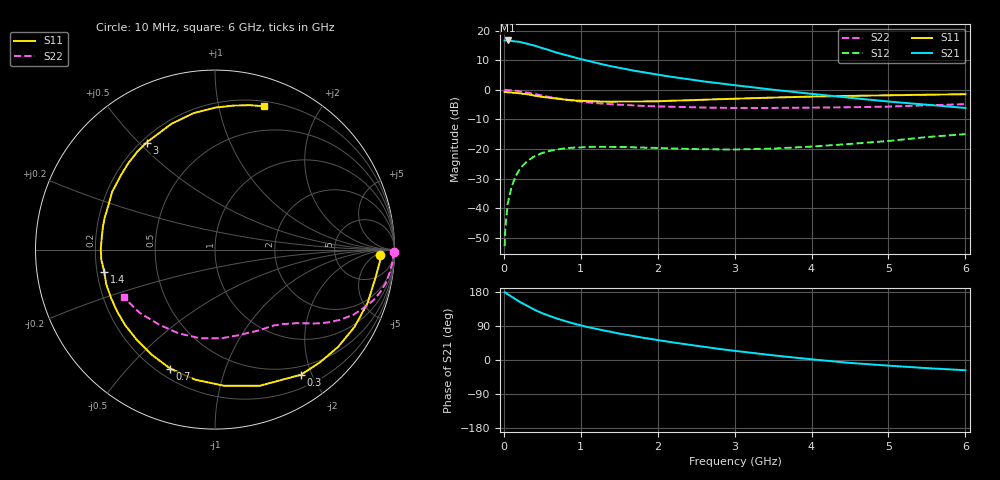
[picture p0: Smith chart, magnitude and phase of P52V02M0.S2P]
! SIEMENS Small Signal Semiconductors
! BFP183
! Si NPN RF Bipolar Junction Transistor in SOT143
! VCE = 2 V  IC = 2 mA
! Common Emitter S-Parameters:  March  1996
# GHz  S  MA  R  50
!  f  S11  S21  S12  S22
! GHz  MAG  ANG  MAG  ANG  MAG  ANG  MAG  ANG
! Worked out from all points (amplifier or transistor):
!   36 points, 10 MHz to 6 GHz, reference 50 ohm
!   highest |S21| = 16.7 dB at 50 MHz (marker M1)
!   |S21| within 3 dB of that: start of sweep to 554.7 MHz
!   unconditionally stable (mu >= 1): 2.078 GHz to 5.998 GHz
!   at 250 MHz: K = 0.12, MSG = 20.7 dB, |S12| = -25.4 dB
!   at 1.4 GHz: K = 0.68, MSG = 13.6 dB, |S12| = -19.3 dB
!   at 6 GHz: K = 1.00, MSG = 4.4 dB, |S12| = -15.0 dB
!   S11 on the Smith chart (normalised r, x): 10 MHz: 20, -8; 300 MHz: 0.38, -1.84; 700 MHz: 0.25, -0.66; 1.4 GHz: 0.23, -0.09; 3 GHz: 0.22, +0.53; 6 GHz: 0.25, +1.37
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0.01  0.9183 -1.9  6.817 179.0  0.0023 82.7  0.9991 -0.7
0.02  0.9215 -4.0  6.808 178.0  0.0048 85.3  0.9936 -1.5
0.05  0.908 -9.9  6.819 173.6  0.012 87.2  0.9922 -3.7
0.1  0.9007 -19.3  6.692 167.1  0.0229 78.1  0.9815 -7.5
0.2  0.8742 -38.3  6.477 154.3  0.0444 68.9  0.9507 -14.4
0.25  0.8582 -47.1  6.23 148.5  0.0534 64.0  0.9279 -17.6
0.3  0.8459 -55.5  6.009 143.4  0.062 59.3  0.9009 -20.3
0.4  0.7986 -71.8  5.574 132.5  0.0761 51.1  0.8528 -25.2
0.5  0.7602 -86.2  5.067 123.4  0.0861 44.0  0.7993 -29.3
0.6  0.7331 -98.7  4.638 115.8  0.0938 38.1  0.7547 -32.4
0.7  0.7082 -110.6  4.2 108.8  0.0989 33.4  0.7172 -34.9
0.8  0.6836 -121.0  3.883 102.4  0.1032 29.3  0.6854 -36.9
0.9  0.6657 -130.7  3.585 96.7  0.1058 25.9  0.6565 -38.7
1.1  0.6451 -147.8  3.079 86.4  0.1087 20.2  0.6129 -41.9
1.4  0.6292 -168.7  2.496 74.0  0.109 14.0  0.5733 -46.3
1.8  0.6371 168.5  2 59.1  0.1061 10.4  0.536 -51.9
2.2  0.6569 150.8  1.643 46.4  0.1027 8.9  0.518 -58.4
3  0.7081 122.6  1.199 24.2  0.0985 12.6  0.495 -74.4
3.5  0.7409 109.3  1.005 12.3  0.1021 16.8  0.4954 -85.7
4.5  0.7914 89.8  0.735 -7.7  0.1222 22.8  0.5089 -113.3
5.5  0.8275 76.5  0.561 -21.5  0.1598 23.0  0.5482 -140.0
6  0.8442 71.1  0.495 -27.0  0.1788 19.6  0.5737 -152.5
